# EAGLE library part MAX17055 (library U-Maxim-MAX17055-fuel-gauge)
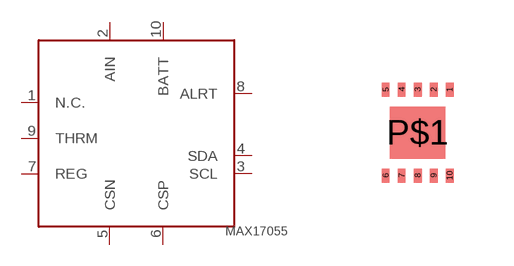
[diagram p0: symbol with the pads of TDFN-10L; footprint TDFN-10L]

Designator prefix U

## MAX17055  [TDFN-10L]
1  N.C.
2  AIN
3  SCL
4  SDA
5  CSN
6  CSP
7  REG
8  ALRT
9  THRM
10  BATT

## Footprint TDFN-10L (pad centres in mm)
TDFN-10L 2.4 X 2.0 X 0.75 mm Exposed Pad Using 0.2 x 0.35 pads
smd 0.2 x 0.35: 1 0.8,1.075; 2 0.4,1.075; 3 0,1.075; 4 -0.4,1.075; 5 -0.8,1.075; 6 -0.8,-1.075; 7 -0.4,-1.075; 8 0,-1.075; 9 0.4,-1.075; 10 0.8,-1.075
smd 1.4 x 1.3: P$1 0,0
